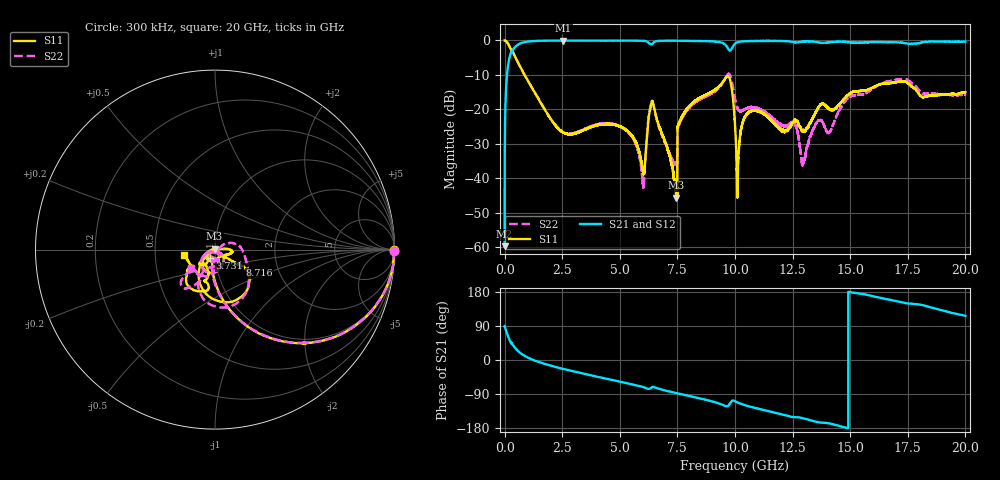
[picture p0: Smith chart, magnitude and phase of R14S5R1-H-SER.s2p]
!{R14S5R1}
!Johanson Technology Inc.
!www.johansontechnology.com
!Test Board Conditions:
!Substrate Type  RO4350B
!Substrate Thickness  20 mil
!Substrate Dk  3.66
!TL Type: GCPW
!TL Trace Width  36 mil
!TL Gap  12 mil
!Electrode orientation  Horizontal
!DUT TOPOLOGY	SERIES
!Mounting Pad LxW  26x36 mil
! Created Wed Nov 25 17:33:21 2020
! 2 Port Network Data from SP1.SP block
! freq  magS11  angS11  magS21  angS21  magS12  angS12  magS22  angS22
# khz S ma R 50
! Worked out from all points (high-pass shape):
!   20001 points, 300 kHz to 20 GHz, reference 50 ohm
!   highest |S21| = -0.03 dB at 2.543 GHz (marker M1); lowest = -59.7 dB at 300 kHz (marker M2)
!   |S21| within 3 dB of the highest: 337.6 MHz to end of sweep
!   lowest |S11| = -45.6 dB at 7.457 GHz (marker M3), VSWR 1.01, Z = 49.8 + j0.462 ohm
!   |S11| at or under -10 dB: 866.6 MHz to end of sweep
!   |S22| runs from -42.7 to 0.0 dB; largest |S21 - S12| = 0.016
!   S11 on the Smith chart (normalised r, x): 300 kHz: open; 3.731 GHz: 0.94, -0.09; 8.716 GHz: 1.30, -0.23; 20 GHz: 0.70, -0.04
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300  0.9987 -0.2  0.001037 89.6  0.0008814 90.1  0.9977 -0.3
110300  0.942 -20.7  0.3332 69.3  0.3341 69.2  0.9413 -20.5
295300  0.7178 -46.6  0.6904 43.2  0.6915 43.2  0.7183 -46.3
2543300  0.04625 -108.1  0.9971 -23.6  0.9958 -23.6  0.04647 -118.1
3334300  0.04836 -115.6  0.9948 -34.9  0.9951 -34.9  0.04951 -133.1
3731300  0.05523 -120.1  0.9946 -40.3  0.9949 -40.3  0.05638 -138.8
5348300  0.04828 -140.0  0.9943 -61.6  0.9931 -61.6  0.04719 -159.8
6000300  0.01276 -109.5  0.9879 -71.2  0.9883 -71.2  0.008322 -120.7
6341300  0.1093 -76.6  0.8837 -74.9  0.8833 -74.9  0.1146 -80.6
6667300  0.06217 -153.7  0.9828 -75.5  0.9831 -75.5  0.05995 -154.9
7457300  0.005218 117.1  0.9929 -87.3  0.9929 -87.3  0.01631 -94.3
7600300  0.06669 -36.4  0.9897 -89.3  0.9912 -89.3  0.06453 29.9
8716300  0.1621 -31.6  0.9775 -104.8  0.9776 -104.8  0.1531 -1.1
9717300  0.3023 -75.7  0.7441 -120.2  0.7449 -120.0  0.3274 -75.0
1.00003e7  0.05964 -142.8  0.8961 -108.6  0.8971 -108.6  0.1445 -118.4
1.01263e7  0.01189 -5.4  0.9463 -112.5  0.9453 -112.5  0.1006 -104.1
1.06063e7  0.09181 -3.5  0.978 -122.5  0.978 -122.4  0.1064 -72.4
1.25563e7  0.06702 -113.5  0.9431 -150.9  0.9452 -150.8  0.06437 -94.3
1.29553e7  0.04953 -144.2  0.9641 -153.9  0.9635 -153.8  0.01681 -88.9
1.33343e7  0.07085 -123.2  0.9668 -160.0  0.9661 -159.9  0.0466 -61.2
1.66673e7  0.2367 -105.5  0.9433 159.6  0.938 159.4  0.2559 -125.0
2e7  0.1779 -169.9  0.9619 116.5  0.9595 116.7  0.1664 -143.1
